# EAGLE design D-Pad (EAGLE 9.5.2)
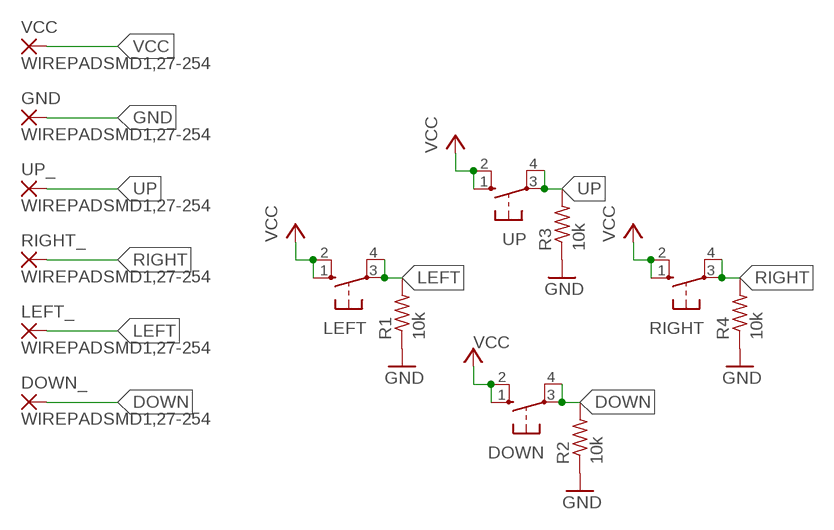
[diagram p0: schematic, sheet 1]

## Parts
DOWN  10-XX  [B3F-10XX]
DOWN_  WIREPADSMD1,27-254  [SMD1,27-2,54]
GND  WIREPADSMD1,27-254  [SMD1,27-2,54]
LEFT  10-XX  [B3F-10XX]
LEFT_  WIREPADSMD1,27-254  [SMD1,27-2,54]
R1  10k  R-US_R0805  [R0805]
R2  10k  R-US_R0805  [R0805]
R3  10k  R-US_R0805  [R0805]
R4  10k  R-US_R0805  [R0805]
RIGHT  10-XX  [B3F-10XX]
RIGHT_  WIREPADSMD1,27-254  [SMD1,27-2,54]
UP  10-XX  [B3F-10XX]
UP_  WIREPADSMD1,27-254  [SMD1,27-2,54]
VCC  WIREPADSMD1,27-254  [SMD1,27-2,54]

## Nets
DOWN: DOWN.3(P) DOWN.4(P1) DOWN_.1(P) R2.2
GND: GND.1(P) R1.1 R2.1 R3.1 R4.1
LEFT: LEFT.3(P) LEFT.4(P1) LEFT_.1(P) R1.2
RIGHT: R4.2 RIGHT.3(P) RIGHT.4(P1) RIGHT_.1(P)
UP: R3.2 UP.3(P) UP.4(P1) UP_.1(P)
VCC: DOWN.1(S) DOWN.2(S1) LEFT.1(S) LEFT.2(S1) RIGHT.1(S) RIGHT.2(S1) UP.1(S) UP.2(S1) VCC.1(P)

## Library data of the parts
DOWN LEFT RIGHT UP = switch-omron:10-XX: OMRON SWITCH; MPN: B3F-1000; OC_FARNELL: 176432; OC_NEWARK: 36M3542
DOWN_ GND LEFT_ RIGHT_ UP_ VCC = wirepad:WIREPAD: Wire PAD connect wire on PCB
R1-R4 = rcl:R-US_: RESISTOR, American symbol; SPICEPREFIX: R

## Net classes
0 default: width 0.305 mm, drill 0.508 mm, clearance 0.254 mm

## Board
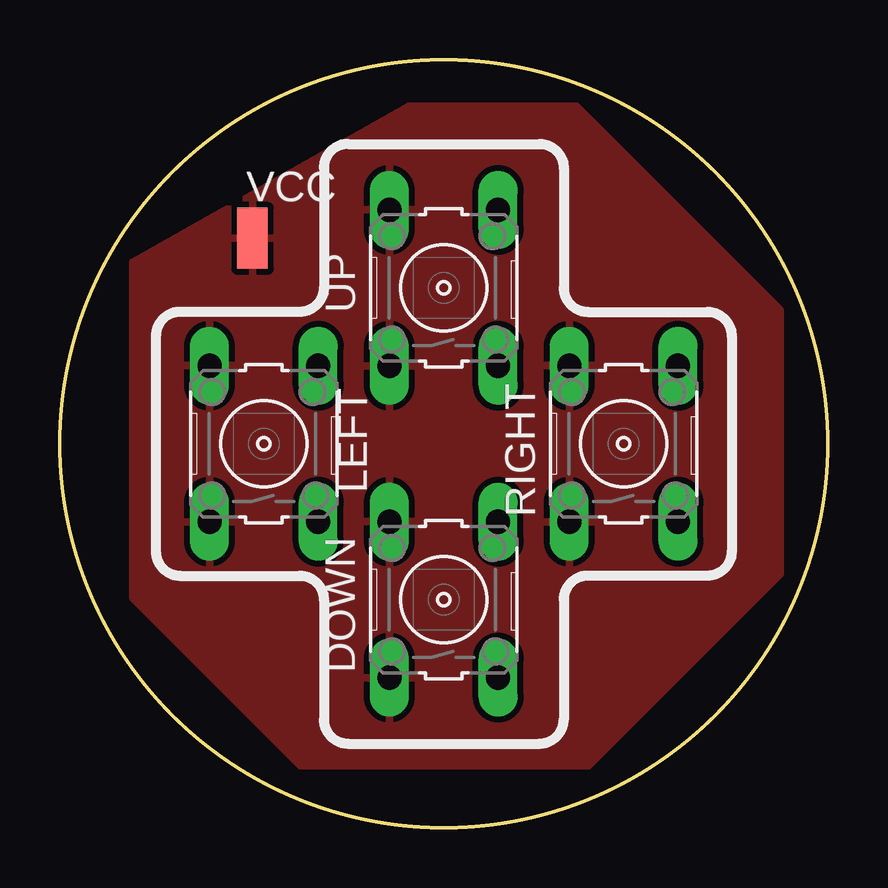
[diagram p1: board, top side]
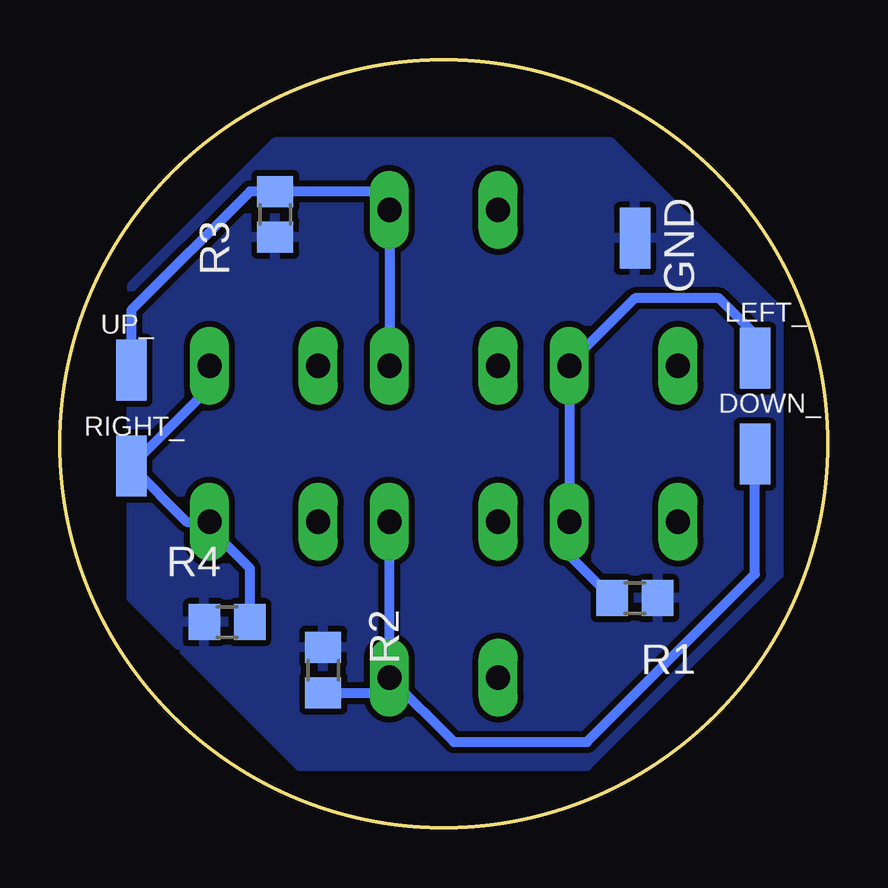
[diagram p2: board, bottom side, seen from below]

Size 32 x 32 mm. Coordinates in mm from the lower left corner, seen from the top.
Outline: circle at 16,16 radius 16
Copper layers (1*16): Top 0.035mm / dielectric 1.5mm / Bottom 0.035mm
Design rules "default *": minimum track width 8mil, minimum drill 20mil, track to track 8mil, track to pad 8mil, pad to pad 8mil, via to via 8mil, smd to smd 8mil, copper to edge 10mil, drill to drill 8mil, minimum pad ring 12mil, minimum via ring 10mil, stop-mask expansion 4mil, vias tented up to drill 25mil, thermal gap 10mil

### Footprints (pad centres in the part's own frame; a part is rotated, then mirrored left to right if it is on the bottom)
B3F-10XX = drill 1.016 long: 1 -3.251,2.261; 2 3.251,2.261; 3 -3.251,-2.261; 4 3.251,-2.261
SMD1,27-2,54 = smd 1.27 x 2.54: 1 0,0
R0805 = smd 1.3 x 1.5: 1 -0.95,0; 2 0.95,0

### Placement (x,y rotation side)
DOWN  16,9.5 90 top
DOWN_  3.03,15.57 180 bottom
GND  8.03,24.57 180 bottom
LEFT  8.5,16 90 top
LEFT_  3.03,19.57 0 bottom
R1  8.03,9.57 180 bottom
R2  21.03,6.57 270 bottom
R3  23.03,25.57 90 bottom
R4  25.03,8.57 0 bottom
RIGHT  23.5,16 90 top
RIGHT_  29.03,15.07 0 bottom
UP  16,22.5 90 top
UP_  29.03,19.07 0 bottom
VCC  8.03,24.57 0 top

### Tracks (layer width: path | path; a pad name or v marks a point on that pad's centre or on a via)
DOWN
  Bottom 0.406: R2.2 18.89,5.62 DOWN.3 | DOWN.3 DOWN.4 | DOWN.3 15.58,3.57 10.03,3.57 3.03,10.57 DOWN_.1
GND
  pour Bottom: 11.03,28.57 23.03,28.57 26.03,25.57 29.03,22.57 29.03,21.57 29.03,9.57 27.03,7.57 22.03,2.57 19.03,2.57 10.03,2.57 2.03,10.57 2.03,21.57 9.03,28.57
LEFT
  Bottom 0.406: R1.2 10.76,11.35 LEFT.3 LEFT.4 10.76,19.34 8.03,22.07 4.53,22.07 3.03,20.57 LEFT_.1
RIGHT
  Bottom 0.406: 26.03,12.75 26.71,12.75 RIGHT_.1 25.76,18.34 RIGHT.4 | 26.03,12.75 RIGHT.3 | R4.2 24.08,10.8 26.03,12.75
UP
  Bottom 0.406: UP_.1 29.03,21.57 24.08,26.52 R3.2 19.03,26.52 UP.4 UP.3
VCC
  pour Top: 14.53,30.07 21.53,30.07 22.03,29.57 30.03,21.57 30.03,10.57 22.03,2.57 10.03,2.57 3.03,9.57 3.03,12.57 3.03,23.57 14.53,30.07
